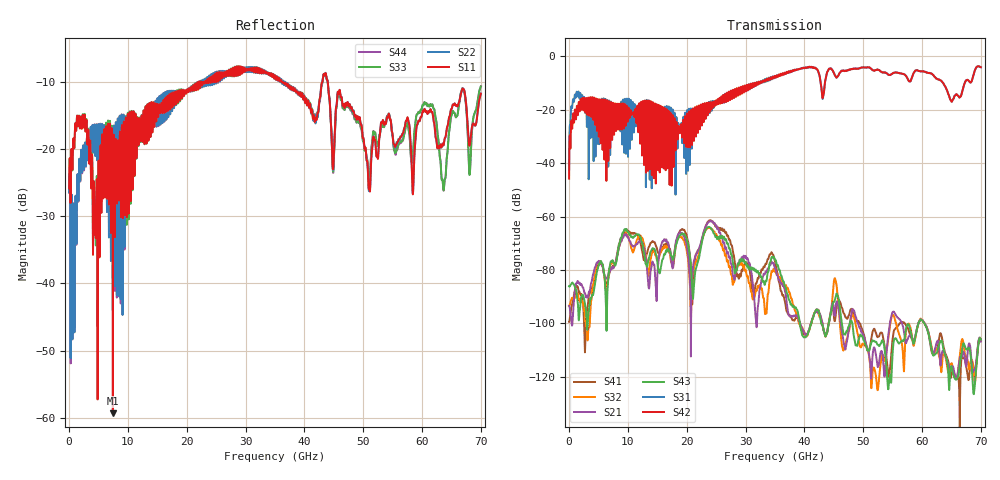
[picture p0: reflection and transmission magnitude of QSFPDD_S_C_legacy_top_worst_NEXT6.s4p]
! AWR Design Environment (8415) Fri Dec 21 09:20:17 2018
! Document = 'CHANNEL TEST'
! nPorts: 4, nXvals: 7001
# HZ S DB R 50
!Freq DBS11 AngS11 DBS12 AngS12 DBS13 AngS13 DBS14 AngS14
!	DBS21 AngS21 DBS22 AngS22 DBS23 AngS23 DBS24 AngS24
!	DBS31 AngS31 DBS32 AngS32 DBS33 AngS33 DBS34 AngS34
!	DBS41 AngS41 DBS42 AngS42 DBS43 AngS43 DBS44 AngS44
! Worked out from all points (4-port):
!   7000 points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, 10 MHz to 70 GHz, reference 50 ohm
!   strongest paths, dB at 10 MHz, 17.51 GHz, 35.01 GHz, 52.51 GHz, 70 GHz:
!     S42: -45.8, -24.5, -7.4, -5.0, -4.0
!     S31: -42.4, -23.4, -7.5, -5.0, -4.0
!     S43: -86.1, -75.0, -76.2, -108.0, -106.0
!     S21: -93.4, -78.3, -79.3, -116.3, -106.8
!     S32: -93.4, -77.6, -80.6, -124.6, -106.5
!     S41: -99.4, -76.5, -76.9, -105.0, -106.2
!   lowest |S11| = -59.3 dB at 7.44 GHz (marker M1), VSWR 1.00, Z = 50.1 - j0.0606 ohm
!   |S11| at or under -10 dB: start of sweep to 22.09 GHz; 36.3 GHz to 43.07 GHz (6.77 GHz wide, 17.1 % of centre); 43.97 GHz to end of sweep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
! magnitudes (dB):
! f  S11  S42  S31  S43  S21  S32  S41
! 10 MHz  -25.8  -45.8  -42.4  -86.1  -93.4  -93.4  -99.4
! 1.3 GHz  -15.8  -18.9  -13.2  -89.0  -84.9  -89.0  -86.1
! 7.44 GHz  -59.3  -18.1  -18.1  -76.5  -78.9  -77.1  -78.6
! 21.01 GHz  -11.2  -20.8  -19.7  -90.0  -80.6  -82.5  -88.3
! 24.02 GHz  -10.2  -17.2  -17.9  -64.1  -61.6  -64.2  -61.4
! 28.08 GHz  -9.0  -14.6  -13.6  -79.4  -83.6  -84.4  -75.6
! 70 GHz  -11.8  -4.0  -4.0  -106.0  -106.8  -106.5  -106.2
